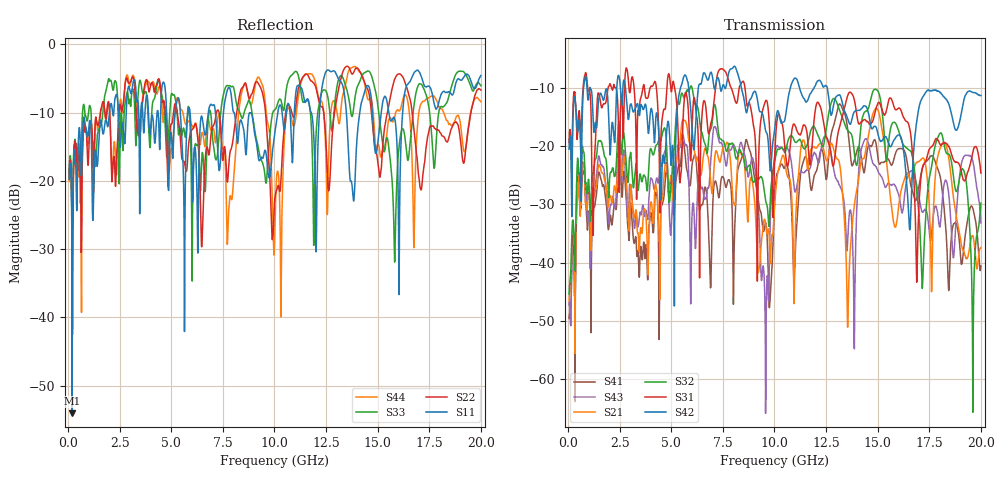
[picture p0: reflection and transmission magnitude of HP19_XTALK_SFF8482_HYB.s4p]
# MHz S MA R 50.00
! FREQ  S11  S12  S13  S14
!  S21  S22  S23  S24
!  S31  S32  S33  S34
!  S41  S42  S43  S44
!  MAG  ANG  MAG  ANG  MAG  ANG  MAG  ANG
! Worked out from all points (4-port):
!   1996 points, 50 MHz to 20 GHz, reference 50 ohm
!   strongest paths, dB at 50 MHz, 5.04 GHz, 10.03 GHz, 15.02 GHz, 20 GHz:
!     S42: -20.5, -20.3, -16.4, -18.0, -11.3
!     S31: -19.3, -9.8, -20.1, -12.6, -24.6
!     S32: -45.4, -24.7, -22.2, -10.6, -29.8
!     S21: -46.5, -27.0, -28.9, -13.9, -37.4
!     S43: -47.3, -31.6, -21.1, -24.3, -33.2
!     S41: -49.6, -26.1, -27.8, -22.2, -40.6
!   lowest |S11| = -54.1 dB at 200 MHz (marker M1), VSWR 1.00, Z = 50.1 + j0.147 ohm
!   |S11| at or under -10 dB: start of sweep to 2 GHz; 5.91 GHz to 6.794 GHz (883.8 MHz wide, 13.9 % of centre); 8.814 GHz to 10.16 GHz (1.347 GHz wide, 14.2 % of centre)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
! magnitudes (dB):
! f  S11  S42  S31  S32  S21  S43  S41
! 50 MHz  -19.8  -20.5  -19.3  -45.4  -46.5  -47.3  -49.6
! 200 MHz  -54.1  -23.2  -19.0  -33.7  -35.5  -36.1  -37.5
! 8.65 GHz  -15.2  -14.3  -12.7  -24.0  -29.5  -23.3  -19.0
! 9.79 GHz  -19.2  -24.1  -19.0  -29.6  -40.1  -33.7  -46.1
! 13.17 GHz  -5.3  -11.3  -16.5  -14.0  -23.4  -26.9  -12.8
! 15.82 GHz  -10.8  -18.8  -13.5  -15.9  -33.8  -26.6  -21.7
! 20 GHz  -4.6  -11.3  -24.6  -29.8  -37.4  -33.2  -40.6
